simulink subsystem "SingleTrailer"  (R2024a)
settings: Solver=VariableStepAuto  StartTime=0.0  StopTime=10.0  RelTol=1e-3
undefined symbols (not defined in the file): D, PlntTraCGHgtAxl, PlntTraDstCGMiddleAxl, PlntTraHtchCxy, PlntTraHtchCz, PlntTraHtchF0z, PlntTraHtchKxy, PlntTraHtchKz, PlntTraInitLatPos, PlntTraInitLatVel, PlntTraInitLongPos, PlntTraInitLongVel, PlntTraInitPitchAng, PlntTraInitPitchRate, PlntTraInitRollAng, PlntTraInitRollRate, PlntTraInitVertPos, PlntTraInitVertVel, PlntTraInitYawAng, PlntTraInitYawRate, PlntTraMass, PlntTraNumWhlFrntAxl, PlntTraPitchMomentInertia, PlntTraRollMomentInertia, PlntTraTrckWdth, PlntTraYawMomentInertia, repmat, Row, vector
libraries: autolibutils x7, sharedtransform x4, vehdynlibeom x2, vehdynlibsuspension x1, matrix_library x1
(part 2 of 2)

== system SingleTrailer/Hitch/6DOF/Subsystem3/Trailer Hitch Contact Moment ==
  Vehicle Psi : Inport
  Trailer Psi : Inport  Port=2
  Constant : Constant  Value=0  SampleTime=-1
  Hitch Contact Yaw Moment : Lookup_n-D  NumberOfTableDimensions=1  LookupTableObject=''  BreakpointsForDimension1=[-1 -.9 -45*pi/180 0 45*pi/180 .9 1]  BreakpointsForDimension1FirstPoint=10  BreakpointsForDimension2FirstPoint=10  BreakpointsForDimension1Spacing=12  BreakpointsForDimension2Spacing=12  IndexSearchMethod=Linear search  Table=[-1e6 -1e6 0 0 0 1e6 1e6]  ExtrapMethod=Clip  DiagnosticForOutOfRangeInput=Error  UseLastTableValue=on  InternalRulePriority=Speed  RndMeth=Simplest
  Subtract : Sum  Inputs=+-
  Vector Concatenate1 : Concatenate  NumInputs=3
  Mh : Outport
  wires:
  Trailer Psi/1 -> Subtract/2
  Subtract/1 -> Hitch Contact Yaw Moment/1
  Vehicle Psi/1 -> Subtract/1
  Hitch Contact Yaw Moment/1 -> Vector Concatenate1/3
  Constant/1 -> Vector Concatenate1/2, Vector Concatenate1/1
  Vector Concatenate1/1 -> Mh/1

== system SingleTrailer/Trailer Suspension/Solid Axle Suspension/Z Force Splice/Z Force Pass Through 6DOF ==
  VehFIn : Inport
  WhlFIn : Inport  Port=2
  Vehicle : Inport  Port=3
  Terminator : Terminator
  VehF : Outport
  WhlF : Outport  Port=2
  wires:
  VehFIn/1 -> VehF/1  "F"
  WhlFIn/1 -> WhlF/1  "F"
  Vehicle/1 -> Terminator/1

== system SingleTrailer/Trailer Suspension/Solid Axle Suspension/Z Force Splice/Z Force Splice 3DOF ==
  VehFIn : Inport
  WhlFIn : Inport  Port=2
  Vehicle : Inport  Port=3
  Bus Selector2 : BusSelector  OutputSignals=BdyFrm.Forces.Tires.FrntTires.Lft.Fz,BdyFrm.Forces.Tires.FrntTires.Rght.Fz
  Constant : Constant  Value=PlntTraMass*9.81/4  SampleTime=-1
  Cont LPF IC : autolibutils/Cont LPF IC  wc=1/0.01  aMode=2  dataType=off
  Gain : Gain  Gain=-1
  Gain1 : Gain  Gain=PlntTraNumWhlFrntAxl/2
  Matrix Concatenate : Concatenate  Mode=Multidimensional array
  Matrix Concatenate1 : Concatenate  Mode=Multidimensional array
  Mux : Mux  Inputs=2
  Reshape : Reshape  OutputDimensionality=Row vector (2-D)
  Selector4 : Selector  NumberOfDimensions=2  InputPortWidth=3  IndexOptions=Index vector (dialog),Select all  Indices=[1 2],1  OutputSizes=1,1
  Selector5 : Selector  NumberOfDimensions=2  InputPortWidth=3  IndexOptions=Index vector (dialog),Select all  Indices=[1 2],1  OutputSizes=1,1
  VehF : Outport
  WhlF : Outport  Port=2
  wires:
  Gain1/1 -> Cont LPF IC/1
  Cont LPF IC/1 -> Reshape/1
  Selector5/1 -> Matrix Concatenate1/1
  Gain/1 -> Matrix Concatenate1/2
  Matrix Concatenate1/1 -> VehF/1  "F"
  VehFIn/1 -> Selector5/1
  Constant/1 -> Cont LPF IC/2
  Reshape/1 -> Gain/1, Matrix Concatenate/2
  Mux/1 -> Gain1/1
  Selector4/1 -> Matrix Concatenate/1
  Vehicle/1 -> Bus Selector2/1
  WhlFIn/1 -> Selector4/1
  Bus Selector2/1 -> Mux/1  "<Fz>"
  Bus Selector2/2 -> Mux/2  "<Fz>"
  Matrix Concatenate/1 -> WhlF/1  "F"

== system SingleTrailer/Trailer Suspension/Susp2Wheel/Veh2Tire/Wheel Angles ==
  SteerAng : Inport
  SteerCmb : Inport  Port=2
  Constant3 : Constant  Value=ones(1,2).*0  SampleTime=-1
  Reshape : Reshape  OutputDimensionality=Row vector (2-D)
  Reshape1 : Reshape  OutputDimensionality=Row vector (2-D)
  Reshape2 : Reshape  OutputDimensionality=Row vector (2-D)
  Vector Concatenate3 : Concatenate  NumInputs=3  Mode=Multidimensional array
  "WhlAng " : Outport  VectorParamsAs1DForOutWhenUnconnected=off
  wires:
  SteerAng/1 -> Reshape/1
  Reshape2/1 -> Vector Concatenate3/2
  SteerCmb/1 -> Reshape1/1
  Reshape1/1 -> Vector Concatenate3/1
  Reshape/1 -> Vector Concatenate3/3
  Vector Concatenate3/1 -> "WhlAng "/1
  Constant3/1 -> Reshape2/1

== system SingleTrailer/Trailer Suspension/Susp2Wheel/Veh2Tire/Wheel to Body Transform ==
  VelVeh : Inport  Partition=on  PartitionDimension=2  PartitionWidth=1  PartitionOffset=0
  WheelAngles : Inport  Port=2  Partition=on  PartitionDimension=2  PartitionWidth=1  PartitionOffset=0
  Constant : Constant  Value=[pi;0;0]  SampleTime=-1
  Demux1 : Demux  Outputs=3
  Divide1 : Product  Inputs=**  Multiplication=Matrix(*)
  Divide2 : Product  Inputs=**  Multiplication=Matrix(*)
  For Each : ForEach  DisableCoverage=on
  Rotation Angles to Direction Cosine Matrix : sharedtransform/Rotation Angles to Direction Cosine Matrix  rotationOrder=ZYX  aMode=2
  Rotation Angles to Direction Cosine Matrix1 : sharedtransform/Rotation Angles to Direction Cosine Matrix  rotationOrder=ZYX  aMode=2
  Selector : Selector  InputPortWidth=3  IndexOptions=Index vector (dialog)  Indices=[3 2 1]  OutputSizes=1
  Selector1 : Selector  InputPortWidth=3  IndexOptions=Index vector (dialog)  Indices=[3 2 1]  OutputSizes=1
  xdotWheel : Outport  ConcatenationDimension=1  VectorParamsAs1DForOutWhenUnconnected=off
  ydotWheel : Outport  Port=2  ConcatenationDimension=1  VectorParamsAs1DForOutWhenUnconnected=off
  zdotWheel : Outport  Port=3  ConcatenationDimension=1  VectorParamsAs1DForOutWhenUnconnected=off
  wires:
  Constant/1 -> Selector1/1
  Divide1/1 -> Divide2/2
  Rotation Angles to Direction Cosine Matrix1/1 -> Divide2/1
  Selector1/1 -> Rotation Angles to Direction Cosine Matrix1/1
  Selector/1 -> Rotation Angles to Direction Cosine Matrix/1
  WheelAngles/1 -> Selector/1
  VelVeh/1 -> Divide1/2
  Rotation Angles to Direction Cosine Matrix/1 -> Divide1/1
  Demux1/3 -> zdotWheel/1
  Demux1/2 -> ydotWheel/1
  Demux1/1 -> xdotWheel/1
  Divide2/1 -> Demux1/1
